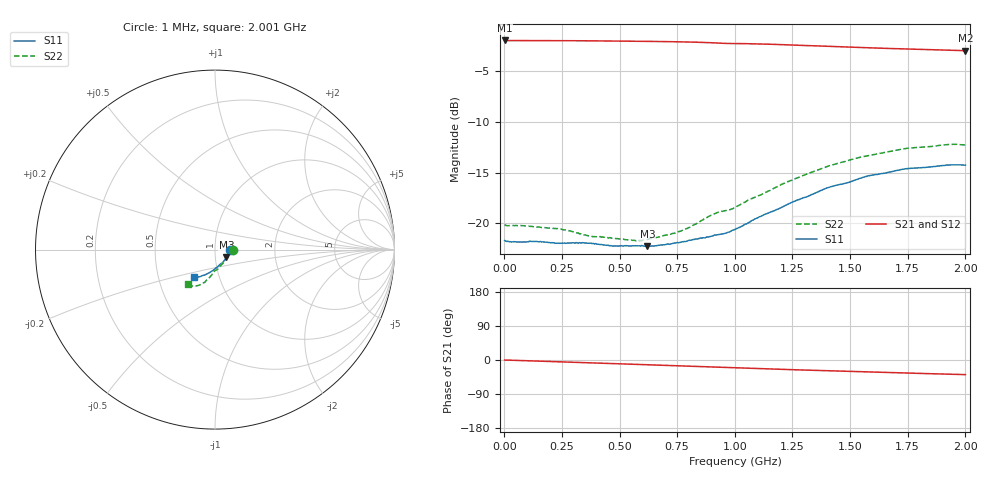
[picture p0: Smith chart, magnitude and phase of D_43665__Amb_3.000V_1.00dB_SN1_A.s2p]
! device id: 43665_
! dir: \\malibu\benchdata\1_engineers\tn_data\43665_75ohm\new\sparar\43665_\amb\3p000v\1p00db
! Serial: 1
! Insertion: A
! Temp: Amb
! VDD: 3.000V
! Attenuation Step: 1.00dB
! IDD: 1.454241e+00mA
! FILE NAME
! DATE 03-27-2009 08:33:37
! CORRECTED  DATA
#  Hz  S  RI  R  75
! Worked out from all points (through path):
!   401 points, 1 MHz to 2.001 GHz, reference 75 ohm
!   highest |S21| = -1.94 dB at 1 MHz (marker M1); lowest = -2.9 dB at 2.001 GHz (marker M2)
!   group delay of S21, straight-line fit = 54.8 ps
!   lowest |S11| = -22.3 dB at 621 MHz (marker M3), VSWR 1.17, Z = 84.8 - j7.48 ohm
!   |S11| at or under -10 dB: start of sweep to end of sweep
!   |S22| runs from -21.8 to -12.2 dB; largest |S21 - S12| = 0.0048
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1000000  0.082 -0.0011  0.8003 -0.00117  0.8006 -0.00138  0.0983 -0.00139
2.36e8  0.0788 -0.011  0.7957 -0.0651  0.7959 -0.0655  0.0917 -0.0185
3.36e8  0.078 -0.0174  0.7919 -0.0929  0.7921 -0.0932  0.0842 -0.0267
3.86e8  0.0766 -0.021  0.7895 -0.1064  0.7895 -0.1069  0.0794 -0.032
4.66e8  0.0721 -0.0275  0.7849 -0.1291  0.785 -0.1297  0.0731 -0.0416
5.61e8  0.0676 -0.0373  0.7777 -0.1558  0.7776 -0.1561  0.0623 -0.0537
6.21e8  0.0631 -0.0439  0.7728 -0.1718  0.7726 -0.1723  0.0552 -0.0617
6.71e8  0.0592 -0.0502  0.7686 -0.1859  0.7683 -0.1861  0.0499 -0.0692
7.71e8  0.0497 -0.0636  0.7577 -0.214  0.7576 -0.2141  0.0359 -0.0844
9.16e8  0.0282 -0.0825  0.7353 -0.2528  0.7357 -0.2526  0.0132 -0.111
9.56e8  0.0238 -0.0857  0.7288 -0.2599  0.7291 -0.2597  0.00394 -0.115
1.001e9  0.0195 -0.091  0.7245 -0.2691  0.725 -0.2692  -0.00208 -0.1193
1.096e9  0.00256 -0.1058  0.7114 -0.2926  0.712 -0.2928  -0.0128 -0.1347
1.211e9  -0.0172 -0.1195  0.6929 -0.3197  0.6939 -0.3205  -0.0289 -0.1542
1.336e9  -0.04 -0.1328  0.6704 -0.3443  0.6714 -0.3454  -0.0486 -0.1723
1.406e9  -0.0534 -0.14  0.6574 -0.3585  0.6584 -0.3603  -0.0579 -0.1825
1.491e9  -0.0668 -0.1437  0.6421 -0.3721  0.6424 -0.3741  -0.074 -0.19
1.566e9  -0.0802 -0.1495  0.629 -0.3844  0.6291 -0.3872  -0.0845 -0.1969
1.671e9  -0.0942 -0.152  0.6109 -0.4003  0.6097 -0.4031  -0.1016 -0.2016
1.746e9  -0.1029 -0.1549  0.5979 -0.4109  0.5965 -0.4138  -0.1131 -0.2049
1.916e9  -0.1167 -0.1541  0.5703 -0.4331  0.5679 -0.4338  -0.1392 -0.2008
2.001e9  -0.1195 -0.152  0.5572 -0.4441  0.5528 -0.4459  -0.148 -0.1935
